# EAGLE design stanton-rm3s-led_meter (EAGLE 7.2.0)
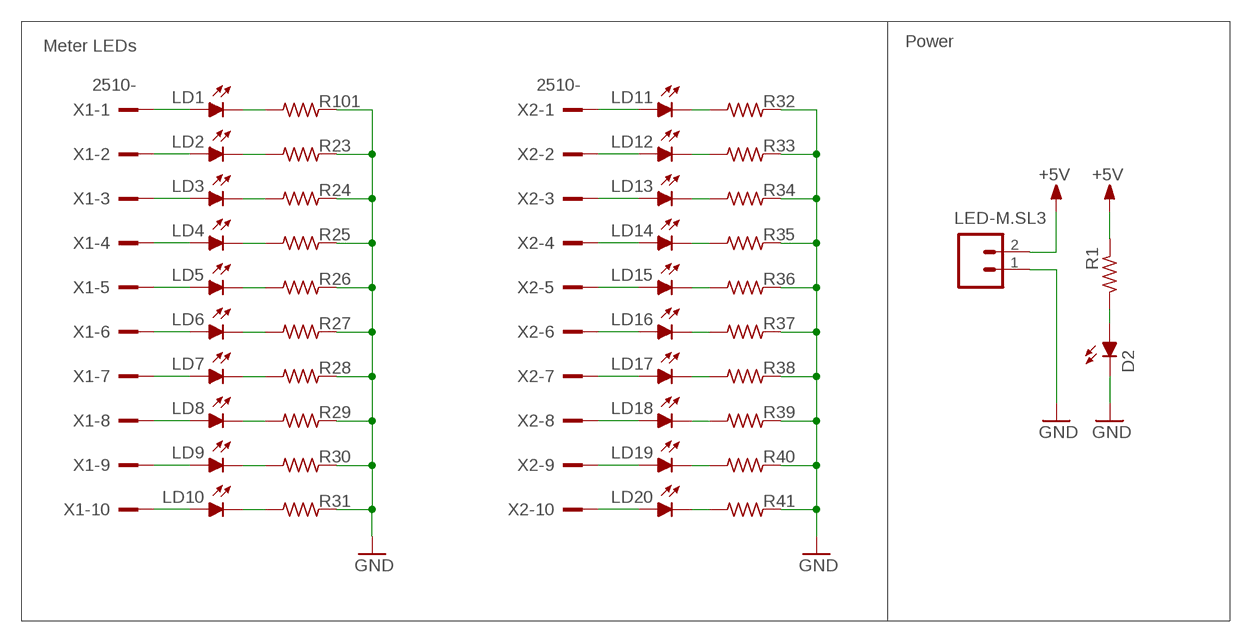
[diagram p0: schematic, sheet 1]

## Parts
D2  LED5MM  [LED5MM]
LD1  LEDSQR2X5  [LED2X5]
LD2  LEDSQR2X5  [LED2X5]
LD3  LEDSQR2X5  [LED2X5]
LD4  LEDSQR2X5  [LED2X5]
LD5  LEDSQR2X5  [LED2X5]
LD6  LEDSQR2X5  [LED2X5]
LD7  LEDSQR2X5  [LED2X5]
LD8  LEDSQR2X5  [LED2X5]
LD9  LEDSQR2X5  [LED2X5]
LD10  LEDSQR2X5  [LED2X5]
LD11  LEDSQR2X5  [LED2X5]
LD12  LEDSQR2X5  [LED2X5]
LD13  LEDSQR2X5  [LED2X5]
LD14  LEDSQR2X5  [LED2X5]
LD15  LEDSQR2X5  [LED2X5]
LD16  LEDSQR2X5  [LED2X5]
LD17  LEDSQR2X5  [LED2X5]
LD18  LEDSQR2X5  [LED2X5]
LD19  LEDSQR2X5  [LED2X5]
LD20  LEDSQR2X5  [LED2X5]
LED-M.SL3  M02  [02P]
R1  R-US_0207/10B  [0207/10B]
R23  R-EU_R1206  [R1206]
R24  R-EU_R1206  [R1206]
R25  R-EU_R1206  [R1206]
R26  R-EU_R1206  [R1206]
R27  R-EU_R1206  [R1206]
R28  R-EU_R1206  [R1206]
R29  R-EU_R1206  [R1206]
R30  R-EU_R1206  [R1206]
R31  R-EU_R1206  [R1206]
R32  R-EU_R1206  [R1206]
R33  R-EU_R1206  [R1206]
R34  R-EU_R1206  [R1206]
R35  R-EU_R1206  [R1206]
R36  R-EU_R1206  [R1206]
R37  R-EU_R1206  [R1206]
R38  R-EU_R1206  [R1206]
R39  R-EU_R1206  [R1206]
R40  R-EU_R1206  [R1206]
R41  R-EU_R1206  [R1206]
R101  R-EU_R1206  [R1206]
X1  2510-  [PAK100/2500-10]
X2  2510-  [PAK100/2500-10]

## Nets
+5V: LED-M.SL3.2 R1.1
GND: D2.K(C) LED-M.SL3.1 R23.2 R24.2 R25.2 R26.2 R27.2 R28.2 R29.2 R30.2 R31.2 R32.2 R33.2 R34.2 R35.2 R36.2 R37.2 R38.2 R39.2 R40.2 R41.2 R101.2
N$1: D2.A R1.2
N$7: LD1.K(C) R101.1
N$10: LD2.K(C) R23.1
N$11: LD3.K(C) R24.1
N$12: LD4.K(C) R25.1
N$13: LD5.K(C) R26.1
N$14: LD6.K(C) R27.1
N$15: LD7.K(C) R28.1
N$16: LD8.K(C) R29.1
N$17: LD9.K(C) R30.1
N$18: LD10.K(C) R31.1
N$19: LD1.A X1.1
N$20: LD2.A X1.2
N$21: LD3.A X1.3
N$22: LD4.A X1.4
N$23: LD5.A X1.5
N$24: LD6.A X1.6
N$25: LD7.A X1.7
N$26: LD8.A X1.8
N$27: LD9.A X1.9
N$29: LD10.A X1.10
N$30: LD11.A X2.1
N$32: LD12.A X2.2
N$33: LD13.A X2.3
N$34: LD14.A X2.4
N$35: LD15.A X2.5
N$36: LD16.A X2.6
N$37: LD17.A X2.7
N$38: LD18.A X2.8
N$39: LD19.A X2.9
N$40: LD20.A X2.10
N$41: LD11.K(C) R32.1
N$42: LD12.K(C) R33.1
N$43: LD13.K(C) R34.1
N$44: LD14.K(C) R35.1
N$45: LD15.K(C) R36.1
N$46: LD16.K(C) R37.1
N$47: LD17.K(C) R38.1
N$48: LD18.K(C) R39.1
N$49: LD19.K(C) R40.1
N$50: LD20.K(C) R41.1

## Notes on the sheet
- Meter LEDs | Power

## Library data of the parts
D2 LD1-LD20 = led:LED: LED
LED-M.SL3 = con-amp-quick:M02: AMP QUICK CONNECTOR
R1 = rcl:R-US_: RESISTOR, American symbol
R23-R41 R101 = rcl:R-EU_: RESISTOR, European symbol
X1 X2 = con-3m:2510-: 3M (TM) Pak 100 4-Wall Header Source: 3M

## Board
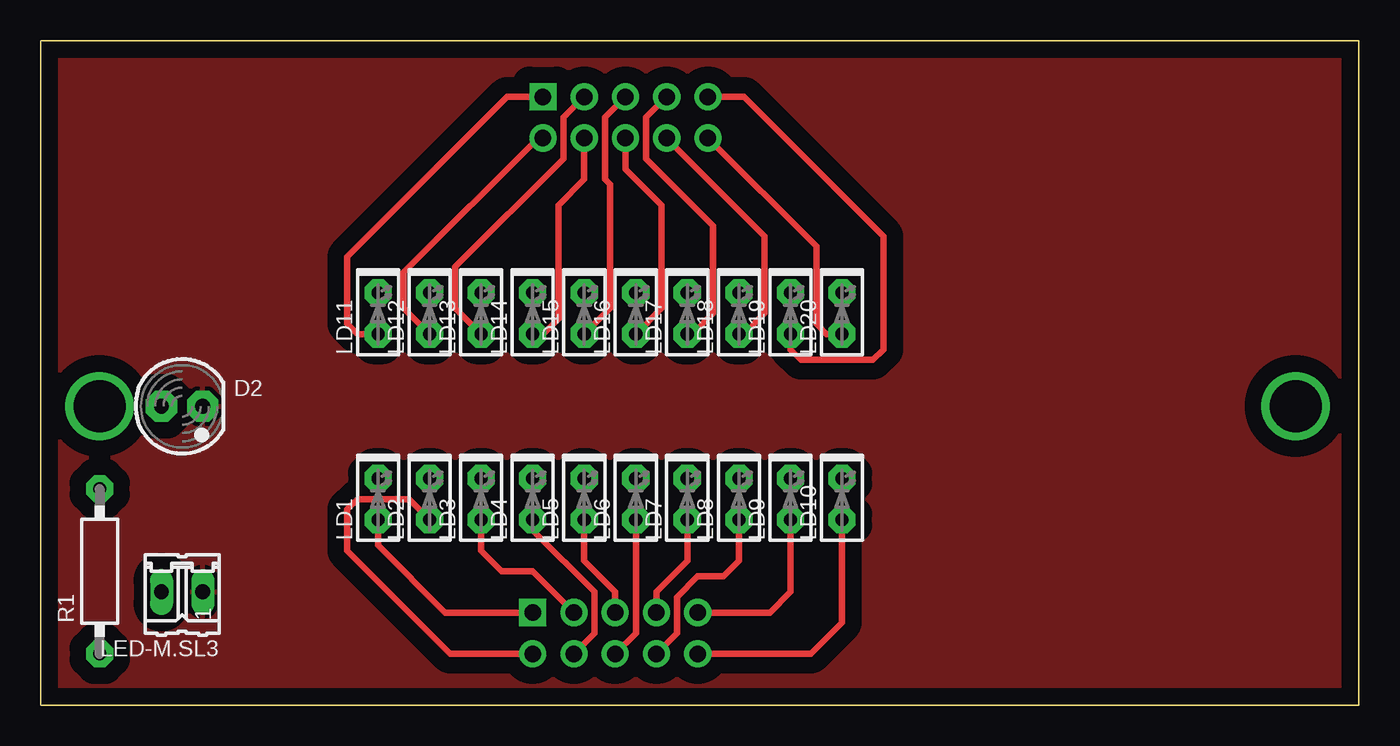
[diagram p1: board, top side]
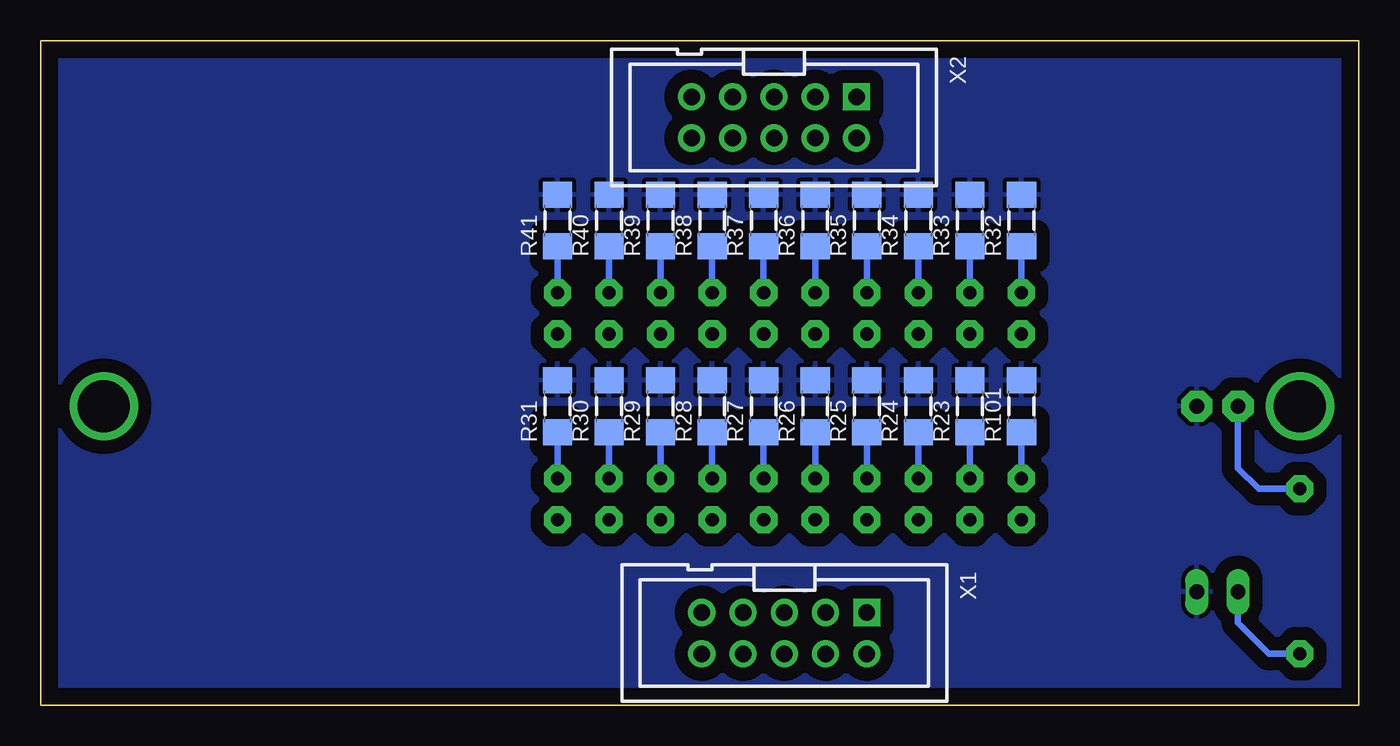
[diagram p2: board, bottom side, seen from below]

Size 81.19 x 40.92 mm. Coordinates in mm from the lower left corner, seen from the top.
Outline: 0,40.92 81.19,40.92 81.19,0 0,0 0,40.92
Copper layers (1*16): Top 0.035mm / dielectric 1.5mm / Bottom 0.035mm
Design rules "default": minimum track width 10mil, minimum drill 24mil, track to track 8mil, track to pad 8mil, pad to pad 8mil, via to via 8mil, smd to smd 8mil, copper to edge 40mil, drill to drill 8mil, minimum pad ring 10mil, minimum via ring 8mil, stop-mask expansion 4mil, vias tented up to drill 0mil, thermal gap 10mil

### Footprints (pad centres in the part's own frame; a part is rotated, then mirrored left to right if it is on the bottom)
LED5MM = drill 0.914 pad 1.93 octagon: A -1.27,0; K 1.27,0
LED2X5 = drill 0.813 pad 1.676 octagon: A -1.27,0; K 1.27,0
02P = drill 0.914 long: 1 -1.27,0; 2 1.27,0
0207/10B = drill 0.813 pad 1.676 octagon: 1 -5.08,0; 2 5.08,0
R1206 = smd 1.6 x 1.803: 1 -1.587,0; 2 1.587,0
PAK100/2500-10 = drill 1.016 pad 1.676 square: 1 -5.08,-1.27 | drill 1.016 pad 1.676: 2 -5.08,1.27; 3 -2.54,-1.27; 4 -2.54,1.27; 5 0,-1.27; 6 0,1.27; 7 2.54,-1.27; 8 2.54,1.27; 9 5.08,-1.27; 10 5.08,1.27

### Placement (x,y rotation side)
D2  8.72,18.41 0 top
LD1  20.78,12.69 90 top
LD2  23.95,12.69 90 top
LD3  27.13,12.69 90 top
LD4  30.31,12.69 90 top
LD5  33.48,12.69 90 top
LD6  36.66,12.69 90 top
LD7  39.83,12.69 90 top
LD8  43,12.69 90 top
LD9  46.18,12.69 90 top
LD10  49.36,12.69 90 top
LD11  20.78,24.12 90 top
LD12  23.95,24.12 90 top
LD13  27.13,24.12 90 top
LD14  30.31,24.12 90 top
LD15  33.48,24.12 90 top
LD16  36.66,24.12 90 top
LD17  39.83,24.12 90 top
LD18  43,24.12 90 top
LD19  46.18,24.12 90 top
LD20  49.36,24.12 90 top
LED-M.SL3  8.72,6.98 180 top
R1  3.63,8.25 90 top
R23  23.95,18.41 90 bottom
R24  27.13,18.41 90 bottom
R25  30.31,18.41 90 bottom
R26  33.48,18.41 90 bottom
R27  36.66,18.41 90 bottom
R28  39.83,18.41 90 bottom
R29  43,18.41 90 bottom
R30  46.18,18.41 90 bottom
R31  49.36,18.41 90 bottom
R32  20.78,29.84 90 bottom
R33  23.95,29.84 90 bottom
R34  27.13,29.84 90 bottom
R35  30.31,29.84 90 bottom
R36  33.48,29.84 90 bottom
R37  36.66,29.84 90 bottom
R38  39.83,29.84 90 bottom
R39  43,29.84 90 bottom
R40  46.18,29.84 90 bottom
R41  49.36,29.84 90 bottom
R101  20.78,18.41 90 bottom
X1  35.38,4.44 180 bottom
X2  36.02,36.19 180 bottom

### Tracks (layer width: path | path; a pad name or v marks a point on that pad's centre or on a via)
+5V
  Bottom 0.406: R1.1 5.54,3.17 7.44,5.07 LED-M.SL3.2
GND
  pour Top (isolate 1.016): 81.11,40.63 0.46,40.63 0.46,0.31 81.11,0.31
  pour Bottom (isolate 0.813): 81.11,40.63 0.46,40.63 0.14,0.31 80.79,0.31
N$1
  Bottom 0.406: D2.A 7.44,14.6 6.18,13.33 R1.2
N$7
  Bottom 0.406: LD1.K R101.1
N$10
  Bottom 0.406: LD2.K R23.1
N$11
  Bottom 0.406: LD3.K R24.1
N$12
  Bottom 0.406: LD4.K R25.1
N$13
  Bottom 0.406: LD5.K R26.1
N$14
  Bottom 0.406: LD6.K R27.1
N$15
  Bottom 0.406: LD7.K R28.1
N$16
  Bottom 0.406: LD8.K R29.1
N$17
  Bottom 0.406: LD9.K R30.1
N$18
  Bottom 0.406: LD10.K R31.1
N$19
  Top 0.406: LD1.A 20.78,9.84 24.91,5.71 X1.1
N$20
  Top 0.406: X1.2 25.23,3.17 18.88,9.52 18.88,12.06 19.51,12.69 22.69,12.69 LD2.A
N$21
  Top 0.406: X1.3 30.31,8.25 28.4,8.25 27.13,9.52 LD3.A
N$22
  Top 0.406: X1.4 34.12,4.44 34.12,6.98 30.31,10.79 LD4.A
N$23
  Top 0.406: X1.5 35.38,6.98 33.48,8.88 LD5.A
N$24
  Top 0.406: X1.6 36.66,4.44 LD6.A
N$25
  Top 0.406: LD7.A 39.83,8.88 37.93,6.98 X1.7
N$26
  Top 0.406: X1.8 39.19,4.44 39.19,6.66 40.47,7.93 42.05,7.93 43,8.88 LD8.A
N$27
  Top 0.406: X1.9 44.91,5.71 46.18,6.98 LD9.A
N$28  (via drill 3.2)
  other vias: 3.63,18.41
N$29
  Top 0.406: X1.10 47.45,3.17 49.36,5.07 LD10.A
N$30
  Top 0.406: X2.1 28.72,37.46 18.88,27.62 18.88,23.49 19.51,22.85 LD11.A
N$31  (via drill 3.2)
  other vias: 77.3,18.41
N$32
  Top 0.406: LD12.A 22.37,24.44 22.37,26.66 30.62,34.92 X2.2
N$33
  Top 0.406: LD13.A 25.54,24.44 25.54,26.98 32.21,33.65 32.21,36.19 X2.3
N$34
  Top 0.406: LD14.A 30.94,22.85 31.89,23.81 31.89,30.79 33.48,32.38 X2.4
N$35
  Top 0.406: LD15.A 35.07,24.44 35.07,32.06 34.75,32.38 34.75,36.19 X2.5
N$36
  Top 0.406: LD16.A 38.24,24.44 38.24,30.79 36.02,33.01 X2.6
N$37
  Top 0.406: X2.7 37.29,36.19 37.29,33.65 41.42,29.52 41.42,24.12 40.15,22.85 LD17.A
N$38
  Top 0.406: LD18.A 43.32,22.85 44.59,24.12 44.59,28.89 X2.8
N$39
  Top 0.406: LD19.A 46.18,21.9 46.81,21.27 51.26,21.27 51.89,21.9 51.89,28.89 43.32,37.46 X2.9
N$40
  Top 0.406: LD20.A 48.4,22.85 47.77,23.49 47.77,28.25 X2.10
N$41
  Bottom 0.406: R32.1 LD11.K
N$42
  Bottom 0.406: LD12.K R33.1
N$43
  Bottom 0.406: LD13.K R34.1
N$44
  Bottom 0.406: LD14.K R35.1
N$45
  Bottom 0.406: LD15.K R36.1
N$46
  Bottom 0.406: LD16.K R37.1
N$47
  Bottom 0.406: LD17.K R38.1
N$48
  Bottom 0.406: LD18.K R39.1
N$49
  Bottom 0.406: LD19.K R40.1
N$50
  Bottom 0.406: LD20.K R41.1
